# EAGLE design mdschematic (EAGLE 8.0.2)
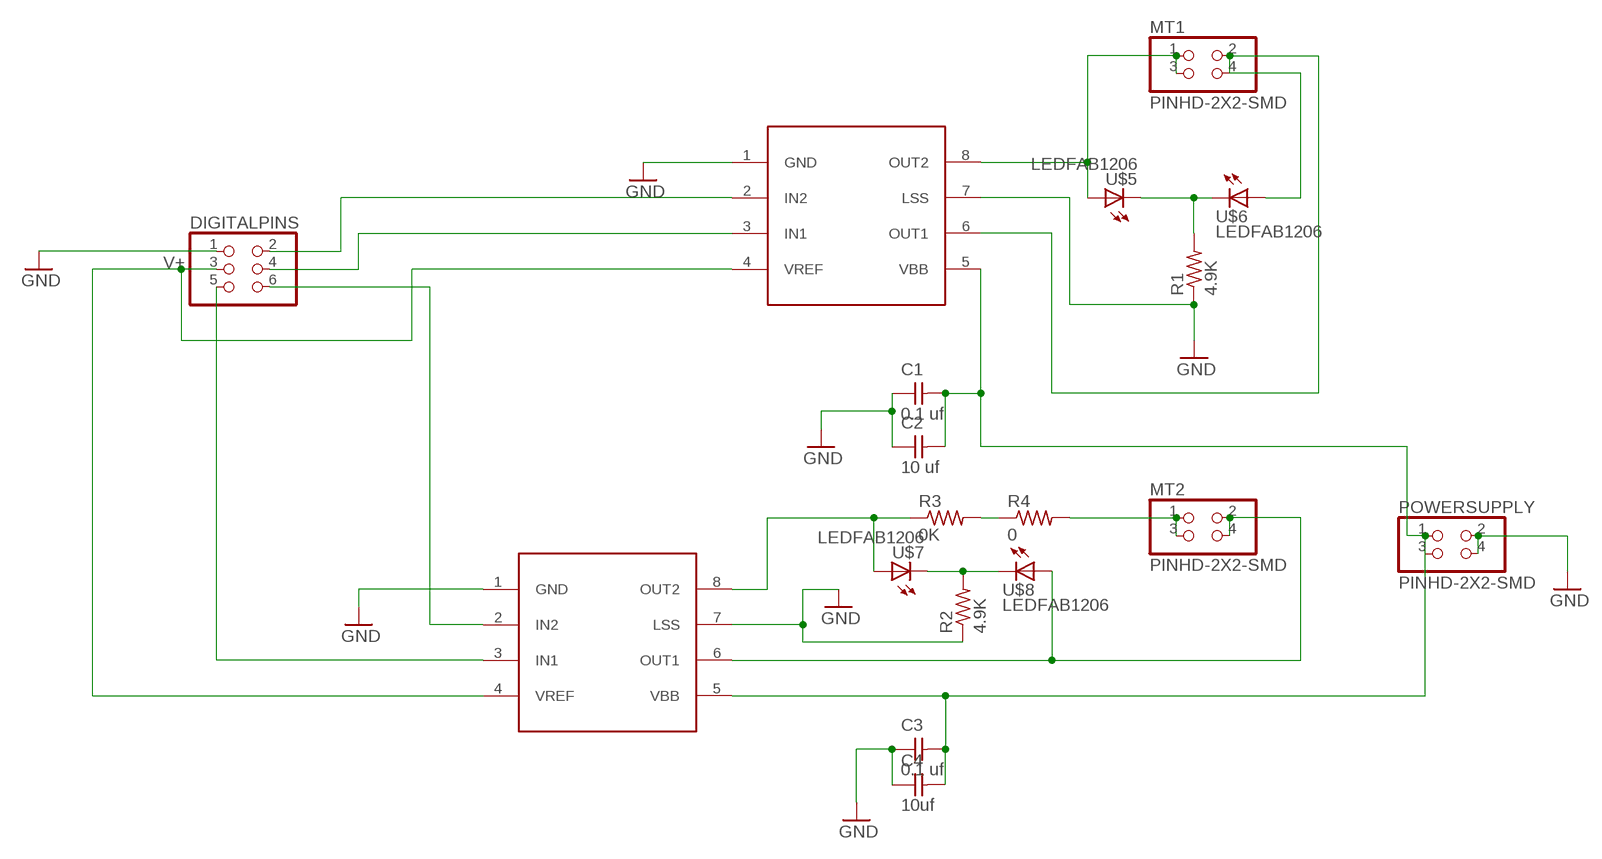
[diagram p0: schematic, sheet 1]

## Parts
C1  0.1 uf  CAP-UNPOLARIZEDFAB  [C1206FAB]
C2  10 uf  CAP-UNPOLARIZEDFAB  [C1206FAB]
C3  0.1 uf  CAP-UNPOLARIZEDFAB  [C1206FAB]
C4  10uf  CAP-UNPOLARIZEDFAB  [C1206FAB]
DIGITALPINS  PINHD-2X3-SMD  [2X03SMD]
MT1  PINHD-2X2-SMD  [2X02SMD]
MT2  PINHD-2X2-SMD  [2X02SMD]
POWERSUPPLY  PINHD-2X2-SMD  [2X02SMD]
R1  4.9K  RES-US1206FAB  [R1206FAB]
R2  4.9K  RES-US1206FAB  [R1206FAB]
R3  0K  RES-US1206FAB  [R1206FAB]
R4  0  RES-US1206FAB  [R1206FAB]
U$1  A4953-H-BRIDGE-MOTOR-DRIVER  [SOIC8]
U$2  A4953-H-BRIDGE-MOTOR-DRIVER  [SOIC8]
U$5  LEDFAB1206  [LED1206FAB]
U$6  LEDFAB1206  [LED1206FAB]
U$7  LEDFAB1206  [LED1206FAB]
U$8  LEDFAB1206  [LED1206FAB]

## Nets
GND: C1.1 C2.1 C3.1 C4.1 DIGITALPINS.1 POWERSUPPLY.2 POWERSUPPLY.4 R1.1 R2.1 U$1.1(GND) U$1.7(LSS) U$2.1(GND) U$2.7(LSS)
N$1: R1.2 U$5.2(C) U$6.2(C)
N$2: R2.2 U$7.2(C) U$8.2(C)
N$3: MT1.1 MT1.3 U$1.8(OUT2) U$5.1(A)
N$4: MT1.2 MT1.4 U$1.6(OUT1) U$6.1(A)
N$5: DIGITALPINS.5 U$2.3(IN1)
N$6: R3.1 U$2.8(OUT2) U$7.1(A)
N$7: MT2.2 MT2.4 U$2.6(OUT1) U$8.1(A)
N$9: MT2.1 MT2.3 R4.2
N$10: R3.2 R4.1
N$11: C1.2 C2.2 C3.2 C4.2 POWERSUPPLY.1 POWERSUPPLY.3 U$1.5(VBB) U$2.5(VBB)
N$14: DIGITALPINS.6 U$2.2(IN2)
N$16: DIGITALPINS.4 U$1.3(IN1)
N$17: DIGITALPINS.2 U$1.2(IN2)
V+: DIGITALPINS.3 U$1.4(VREF) U$2.4(VREF)

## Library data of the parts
C1-C4 = fab:CAP-UNPOLARIZED
DIGITALPINS = fab:PINHD-2X3-SMD: PIN HEADER
MT1 MT2 POWERSUPPLY = fab:PINHD-2X2-SMD
R1-R4 = fab:RES-US: Resistor (US Symbol)
U$1 U$2 = fab:A4953-H-BRIDGE-MOTOR-DRIVER
U$5-U$8 = fab:LED: LED

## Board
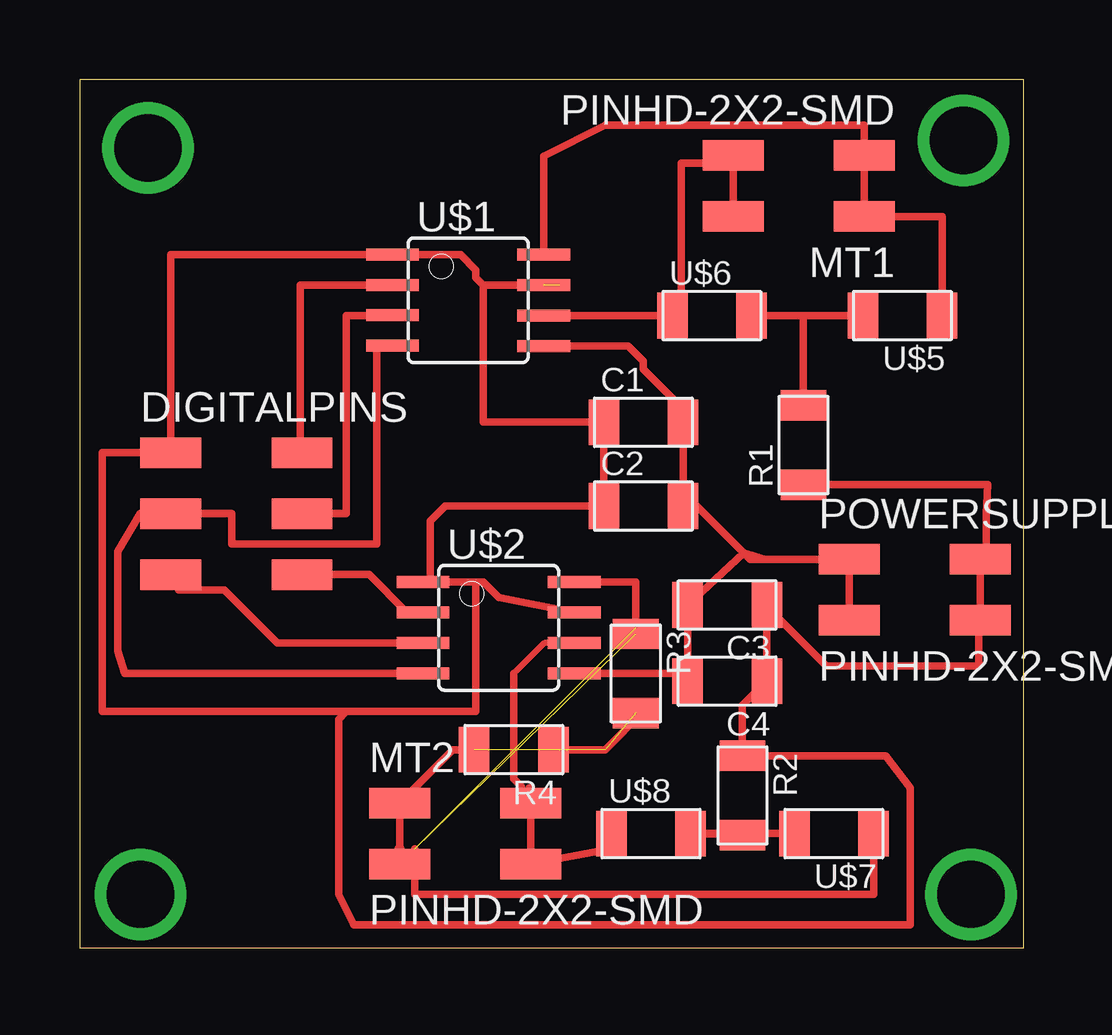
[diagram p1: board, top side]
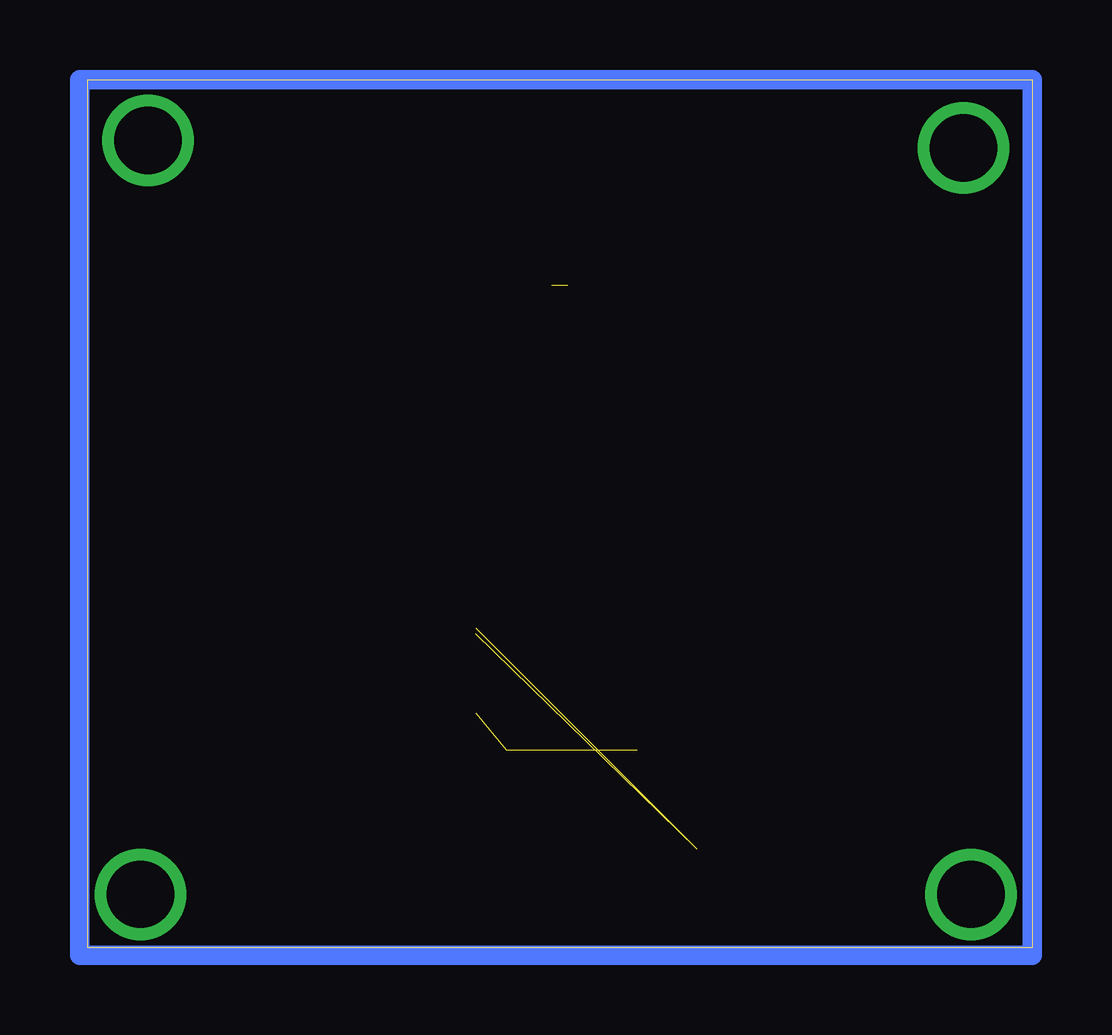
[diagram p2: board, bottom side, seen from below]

Size 39.35 x 36.18 mm. Coordinates in mm from the lower left corner, seen from the top.
Outline: 0,0 39.35,0 39.35,36.18 0,36.18 0,0
Copper layers (1*16): Top 0.035mm / dielectric 1.5mm / Bottom 0.035mm
Design rules "default": minimum track width 10mil, minimum drill 24mil, track to track 8mil, track to pad 8mil, pad to pad 8mil, via to via 8mil, smd to smd 8mil, copper to edge 40mil, drill to drill 8mil, minimum pad ring 10mil, minimum via ring 8mil, stop-mask expansion 4mil, vias tented up to drill 0mil, thermal gap 10mil

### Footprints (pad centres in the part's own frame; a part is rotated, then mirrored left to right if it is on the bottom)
C1206FAB = smd 1.27 x 1.905: 1 -1.651,0; 2 1.651,0
2X03SMD = smd 2.54 x 1.27: 1 -2.54,2.54; 2 2.92,2.54; 3 -2.54,0; 4 2.92,0; 5 -2.54,-2.54; 6 2.92,-2.54
2X02SMD = smd 2.54 x 1.27: 1 -2.54,1.27; 2 2.92,1.27; 3 -2.54,-1.27; 4 2.92,-1.27
R1206FAB = smd 1.27 x 1.905: 1 -1.651,0; 2 1.651,0
SOIC8 = smd 0.5 x 2.2: 1 -1.905,-3.154; 2 -0.645,-3.154; 3 0.625,-3.154; 4 1.895,-3.154; 5 1.905,3.154; 6 0.635,3.154; 7 -0.635,3.154; 8 -1.905,3.154
LED1206FAB = smd 1.27 x 1.905: 1 -1.651,0; 2 1.651,0

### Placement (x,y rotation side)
C1  23.5,21.91 0 top
C2  23.5,18.41 0 top
C3  26.99,14.29 180 top
C4  26.99,11.11 180 top
DIGITALPINS  6.35,18.1 0 top
MT1  30.16,31.75 180 top
MT2  15.88,4.76 0 top
POWERSUPPLY  34.61,14.92 0 top
R1  30.16,20.95 90 top
R2  27.62,6.35 270 top
R3  23.18,11.43 270 top
R4  18.1,8.26 180 top
U$1  16.19,26.99 270 top
U$2  17.46,13.34 270 top
U$5  34.29,26.35 180 top
U$6  26.35,26.35 0 top
U$7  31.43,4.76 180 top
U$8  23.81,4.76 0 top

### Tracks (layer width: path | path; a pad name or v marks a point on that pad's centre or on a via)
GND  (1 unrouted)
  Top 0.305: 16.83,27.62 16.51,27.94 16.51,28.26 15.87,28.89 U$1.1 3.81,28.89 DIGITALPINS.1 0.95,20.64 0.95,9.84 11.11,9.84 | 16.83,27.62 20,27.62 | R1.1 37.85,19.3 37.78,18.1 37.78,16.57 | 37.78,16.19 37.78,16.57 | 37.78,16.57 POWERSUPPLY.2 POWERSUPPLY.4 37.46,13.59 37.46,11.75 31.12,11.75 28.64,14.22 C3.1 C4.1 27.62,10.1 R2.1 33.59,8 34.61,6.67 34.61,0.95 11.43,0.95 10.79,2.22 10.79,9.52 11.11,9.84 | 16.83,27.62 16.83,21.91 C1.1 C2.1 15.24,18.42 14.61,17.78 14.61,15.26 U$2.1 16.51,15.24 | 16.51,15.24 16.83,15.24 17.46,14.6 U$2.7 | 16.51,15.24 16.51,9.84 11.11,9.84
N$1
  Top 0.305: 30.16,26.35 U$6.2 | 30.16,26.35 U$5.2 | R1.2 30.16,26.35
N$2
  Top 0.305: U$8.2 25.34,4.76 R2.2 U$8.2 | U$7.2 U$8.2
N$3
  Top 0.305: U$5.1 35.94,30.48 MT1.1 MT1.3 32.7,34.29 21.91,34.29 19.35,33 U$1.8
N$4
  Top 0.305: MT1.4 MT1.2 27.24,32.7 25.08,32.7 25.08,26.35 U$6.1 U$1.6
N$5
  Top 0.305: U$2.3 8.25,12.71 6.03,14.92 4.13,14.92 DIGITALPINS.5
N$6  (2 unrouted)
  Top 0.305: U$2.8 23.18,15.24 23.18,13.34 | 13.97,4.13 13.97,2.22 33.08,2.22 U$7.1
N$7
  Top 0.254: U$2.6 19.37,12.7 18.1,11.43 | 18.41,6.73 MT2.2
  Top 0.305: 18.73,6.67 MT2.2 MT2.4 22.16,4.13 U$8.1 | 18.1,11.43 18.1,7.05 18.41,6.73
N$8
  Bottom 0.813: 0,36.19 39.69,36.19 39.69,-0.32 0,-0.32 0,36.19
N$9  (1 unrouted)
  Top 0.305: MT2.3 13.33,4.13 MT2.1 15.56,8.26 R4.2 | 21.91,8.26 23.49,9.84
  Top 0.406: MT2.3 13.33,4.13
N$10  (1 unrouted)
  Top 0.305: R4.1 21.91,8.26
N$11
  Top 0.305: POWERSUPPLY.3 POWERSUPPLY.1 28.58,16.19 | 28.58,16.19 27.94,16.19 27.69,16.45 | 27.69,16.45 25.72,18.42 C2.2 C1.2 25.08,21.97 25.08,22.54 23.49,24.13 23.49,24.45 22.86,25.08 U$1.5 | 27.69,16.45 C3.2 C4.2 25.02,11.43 U$2.5 | 27.69,16.45 28.58,16.19
N$12  (via drill 2.8)
  other vias: 2.86,33.34
N$13  (via drill 2.8)
  other vias: 36.83,33.66
N$14
  Top 0.305: U$2.2 13.64,13.98 12.07,15.56 DIGITALPINS.6
N$15  (via drill 2.8)
  other vias: 2.54,2.22
N$16
  Top 0.305: U$1.3 13.04,26.35 11.11,26.35 11.11,18.1 DIGITALPINS.4
N$17
  Top 0.305: DIGITALPINS.2 9.21,20.64 9.21,27.62 13.04,27.62 U$1.2
N$18  (via drill 2.8)
  other vias: 37.15,2.22
V+
  Top 0.305: U$1.4 12.38,25.09 12.38,16.83 6.35,16.83 6.35,18.1 DIGITALPINS.3 2.54,18.1 1.59,16.51 1.59,12.38 1.9,11.44 U$2.4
